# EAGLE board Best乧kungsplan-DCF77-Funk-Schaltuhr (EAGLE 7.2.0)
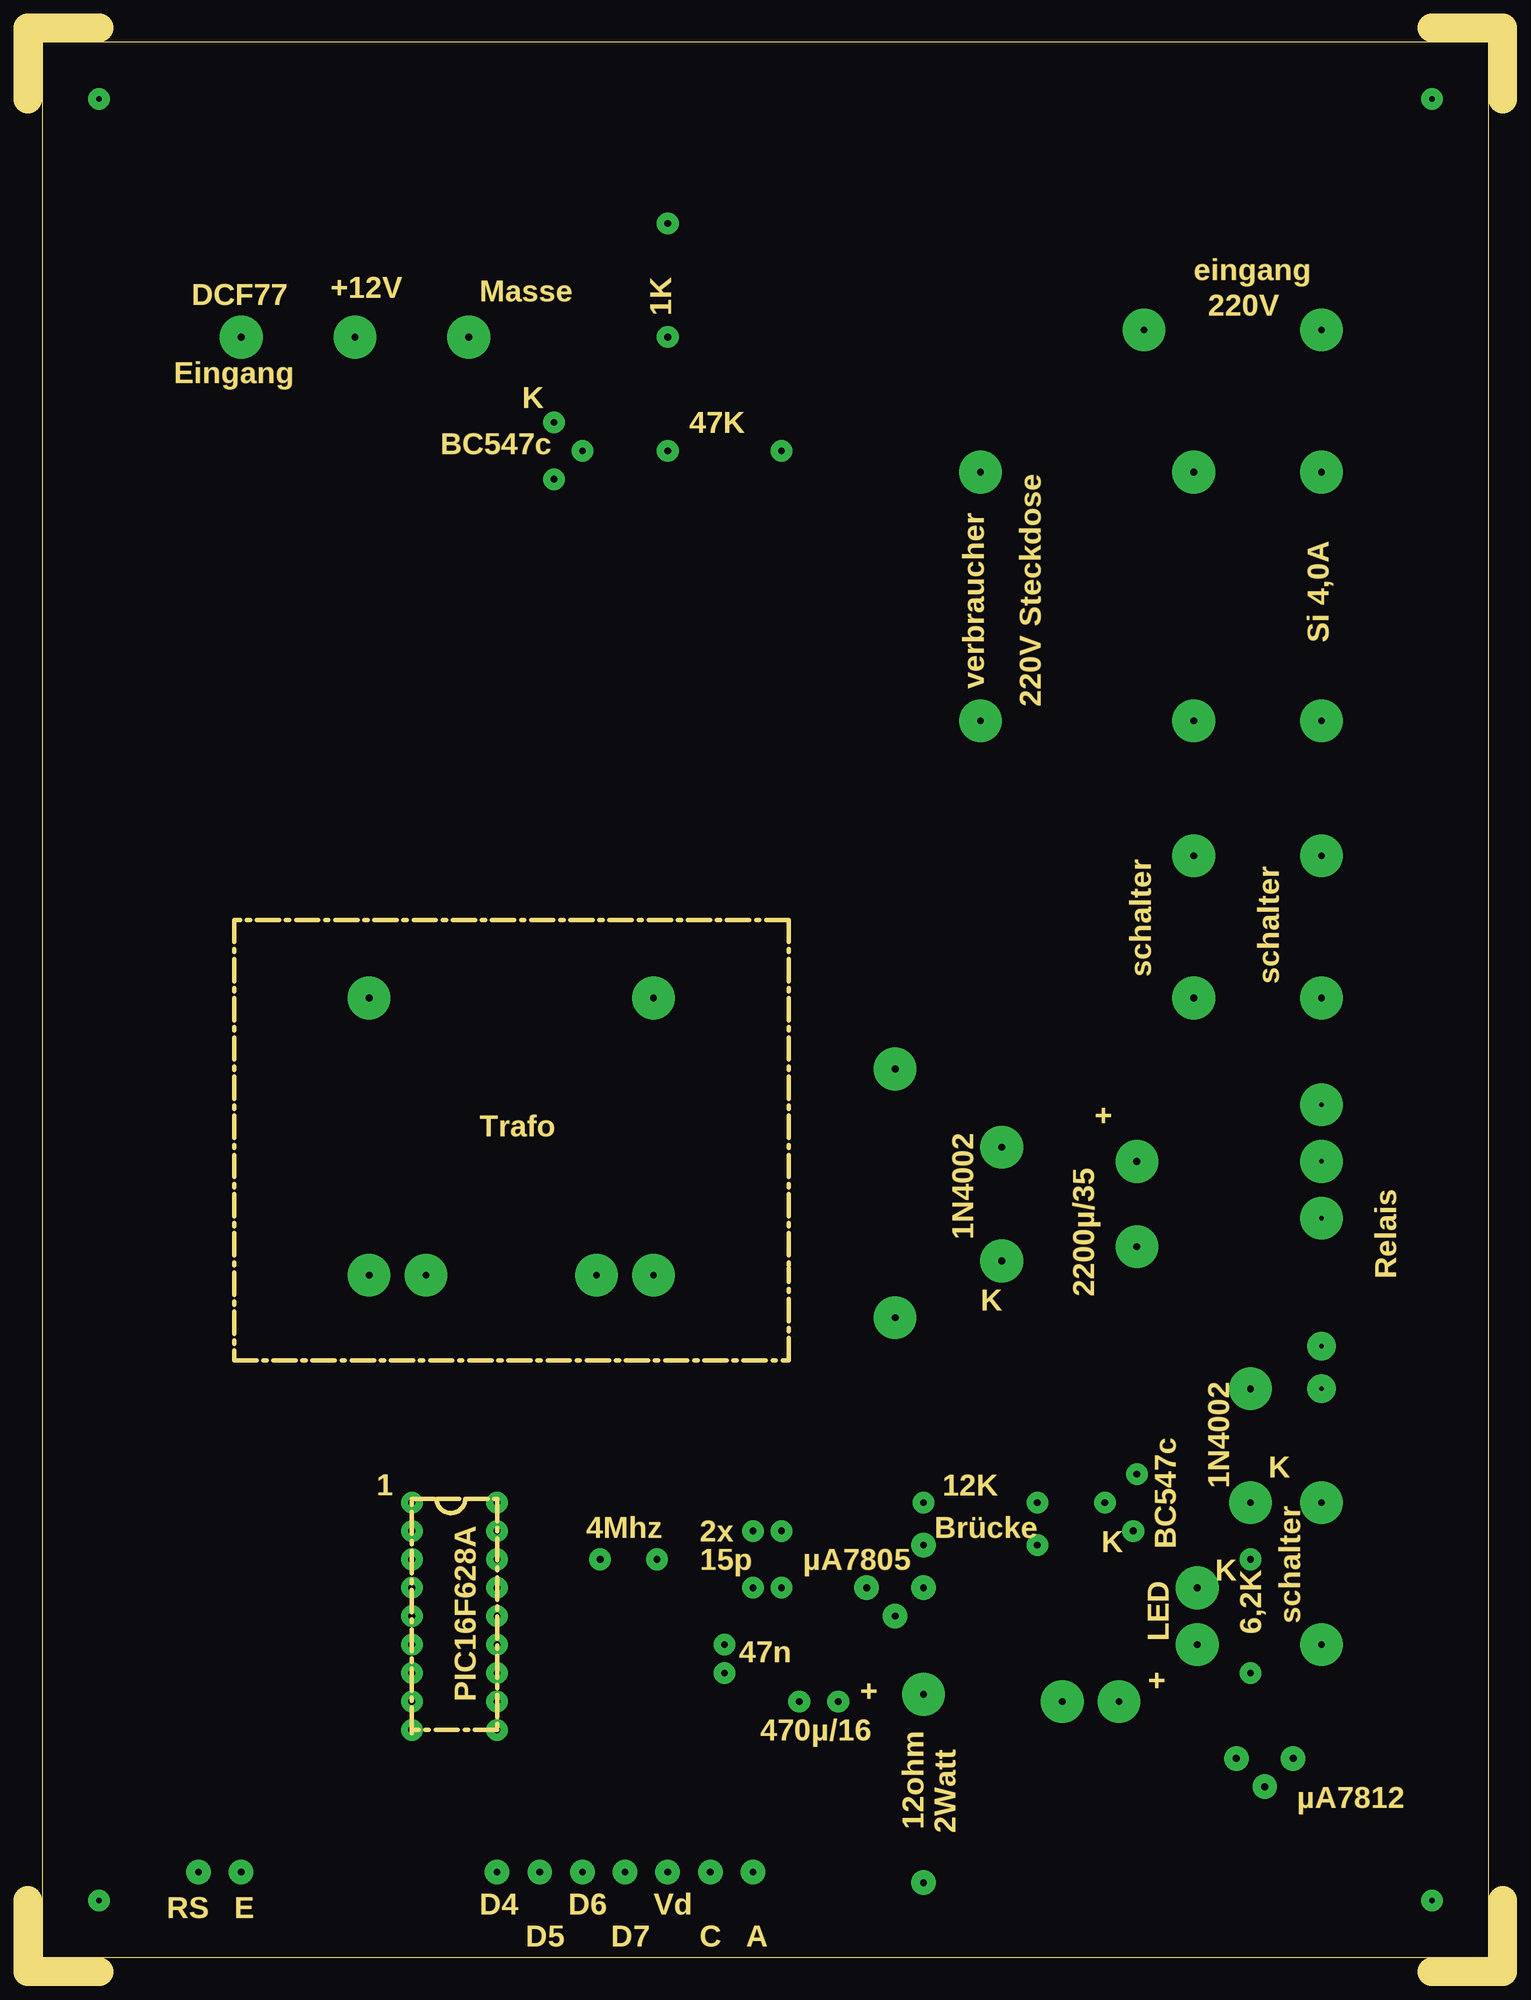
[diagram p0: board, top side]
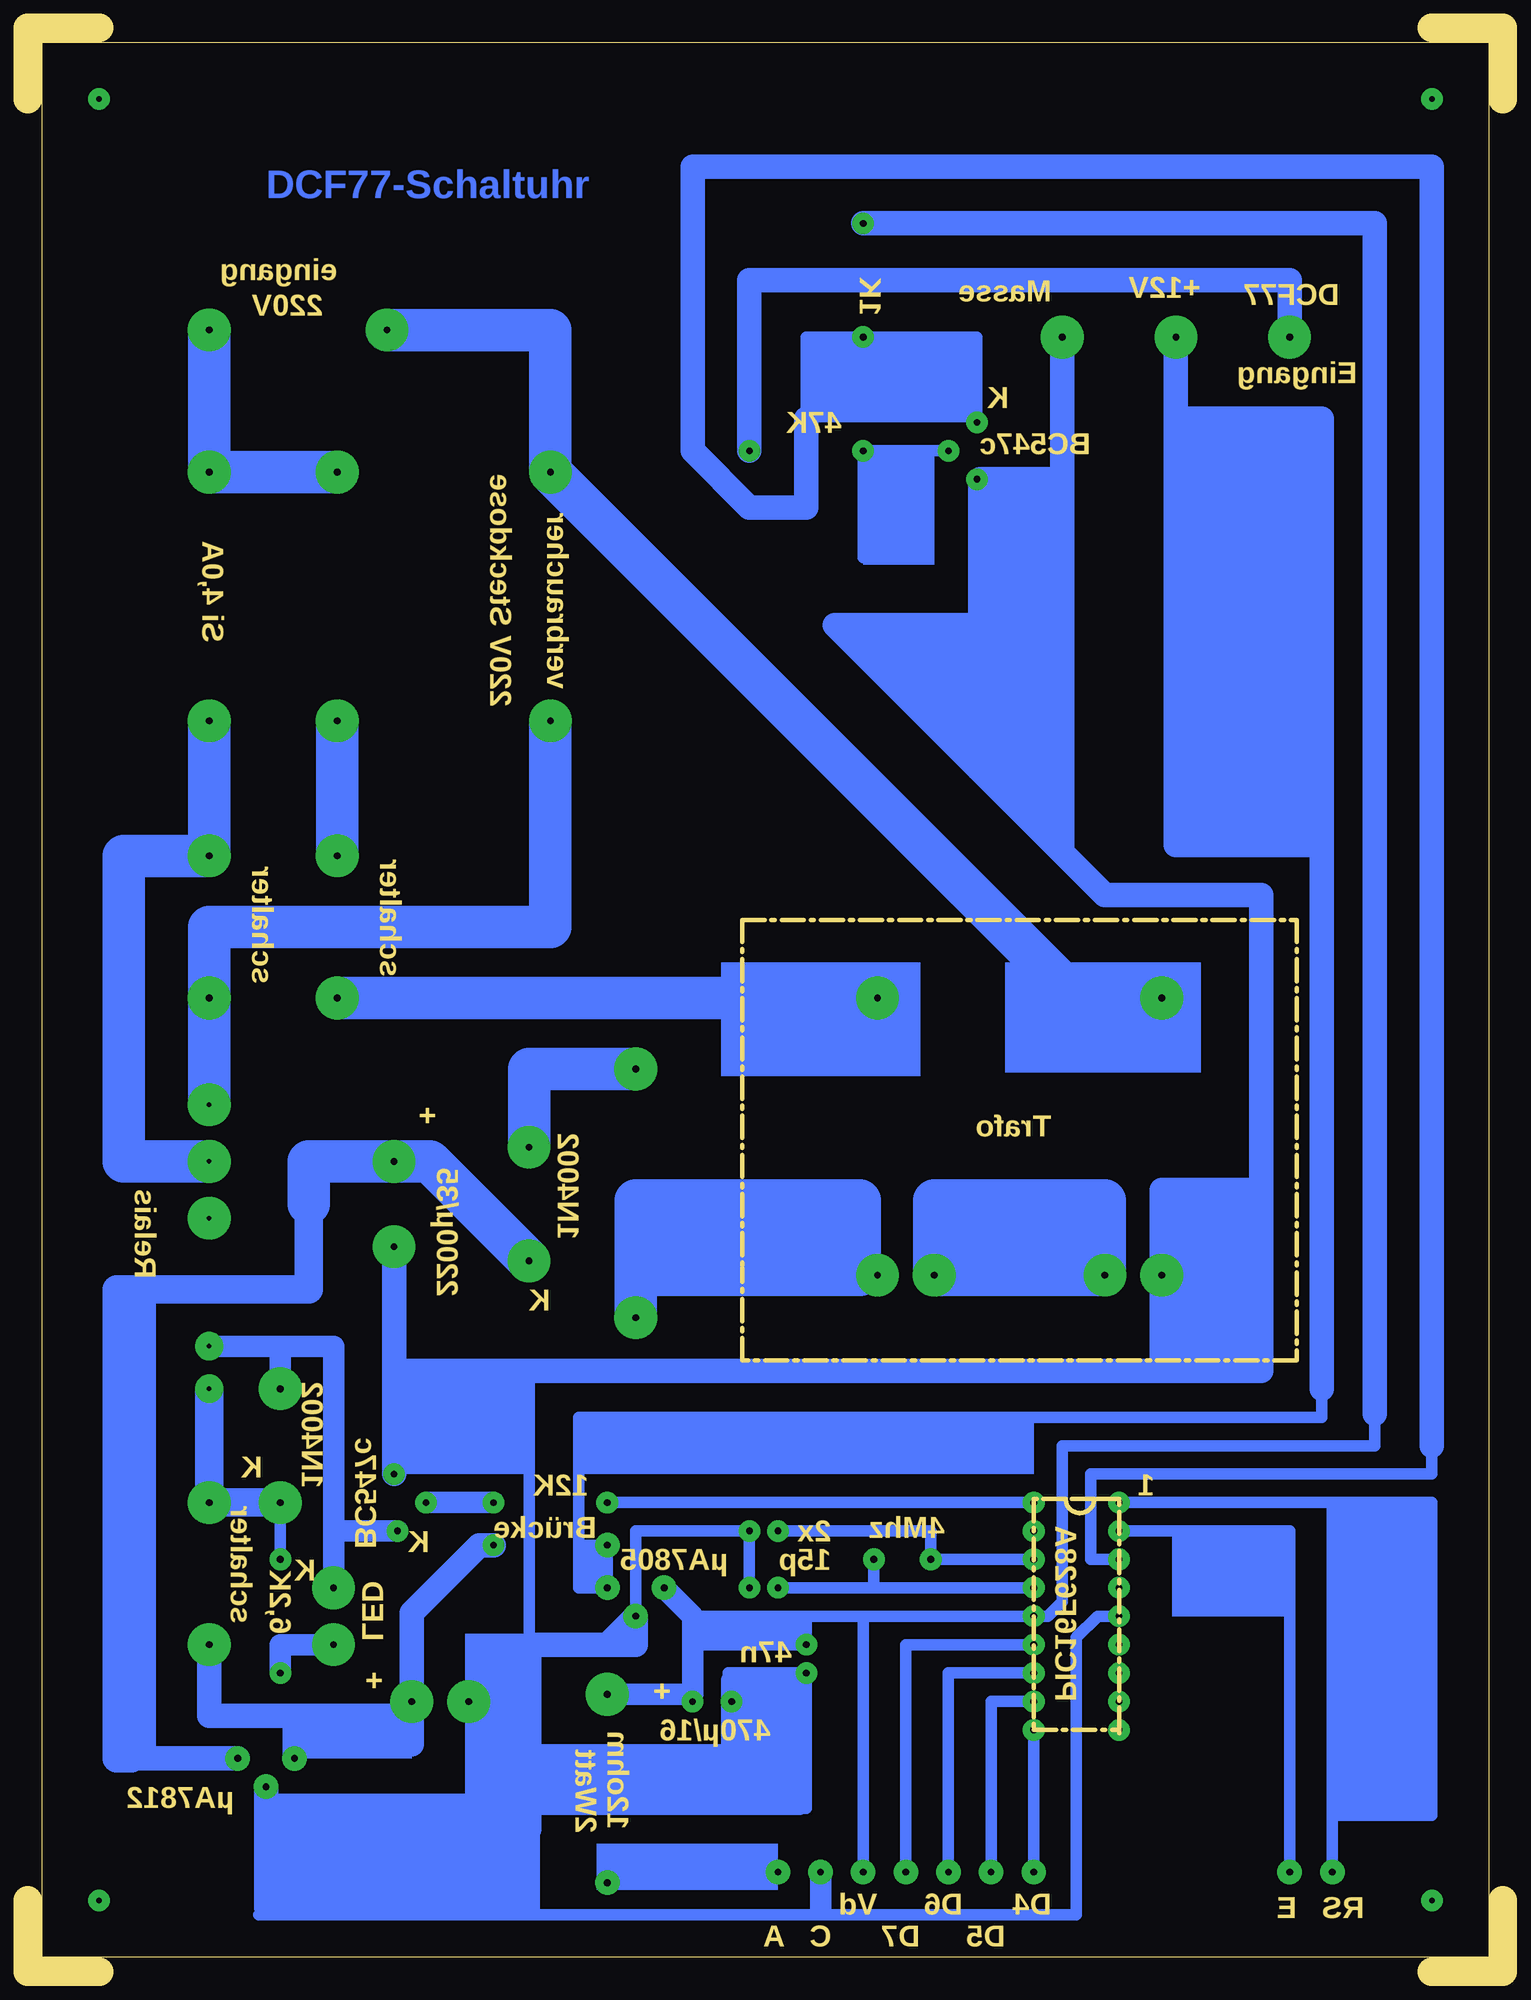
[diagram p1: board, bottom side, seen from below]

Size 131.76 x 173.67 mm. Coordinates in mm from the lower left corner, seen from the top.
Outline: 0,6.35 0,1.59 0,1.27 0,0 6.35,0
Outline: 131.76,6.35 131.76,0 125.41,0
Outline: 0,167.32 0,173.67 6.35,173.67
Outline: 131.76,167.32 131.76,173.67 125.41,173.67
Outline: 36.51,42.23 34.29,42.23 34.29,21.59
Outline: 36.51,42.23 39.05,42.23
Outline: 39.05,42.23 41.91,42.23 41.91,21.59 34.29,21.59
Outline: 34.29,21.59 34.29,21.27
Outline: 36.51,42.23 arc180 39.05,42.23
Outline: 1.27,1.27 130.49,1.27 130.49,172.4 1.27,172.4 1.27,1.27
Outline: 67.94,93.98 67.94,62.87 67.94,62.23 67.94,54.61 18.41,54.61 18.41,93.98 67.94,93.98
Copper layers (1*16): Top 0.035mm / dielectric 1.5mm / Bottom 0.035mm
Design rules "default": minimum track width 10mil, minimum drill 24mil, track to track 8mil, track to pad 8mil, pad to pad 8mil, via to via 8mil, smd to smd 8mil, copper to edge 40mil, drill to drill 8mil, minimum pad ring 10mil, minimum via ring 8mil, stop-mask expansion 4mil, vias tented up to drill 0mil, thermal gap 10mil

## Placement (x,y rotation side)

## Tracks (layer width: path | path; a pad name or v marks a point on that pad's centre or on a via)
S$1  (via drill 0.5 pad 1.93)
  other vias: 6.35,6.35
S$2  (via drill 0.5 pad 1.93)
  other vias: 6.35,167.32
S$3  (via drill 0.5 pad 1.93)
  other vias: 125.41,167.32
S$4  (via drill 0.5 pad 1.93)
  other vias: 125.41,6.35
S$5  (via drill 0.6 pad 1.93)
  other vias: 72.39,24.13
S$6  (via drill 0.6 pad 3.81)
  Bottom 3.81: v35.56,62.23 v50.8,62.23 50.8,68.9 35.56,68.9 v35.56,62.23
S$7  (via drill 0.6 pad 3.81)
  Bottom 3.81: v104.14,111.76 v104.14,99.69
S$8  (via drill 0.6 pad 3.81)
  Bottom 3.81: 77.47,61.91 77.47,62.23 57.47,62.23 57.47,68.9 77.47,68.9 77.47,61.91 | 77.47,61.91 v77.47,58.42
S$9  (via drill 0.6 pad 1.93, 0.6 pad 3.81)
  Bottom 2.184: v19.05,146.05 19.05,151.13 67.31,151.13 v67.31,135.89
S$10  (via drill 0.6 pad 3.81)
  other vias: 104.14,86.99
S$11  (via drill 0.6 pad 3.81)
  Bottom 3.81: v55.88,86.99 103.5,86.99
S$12  (via drill 0.6 pad 1.93, 0.6 pad 2.18, 0.6 pad 3.81)
  Bottom 2.184: v115.57,29.21 115.57,22.86 107.95,22.86 | v97.47,24.13 97.47,32.07 91.44,38.1 v90.17,38.1 | 107.95,22.86 v107.95,19.05 | 107.95,22.86 97.47,22.86 v97.47,24.13 | v97.47,24.13 97.47,20.32
S$13  (via drill 0.4 pad 3.81, 0.6 pad 3.81)
  Bottom 3.81: v85.09,111.76 85.09,93.34 115.57,93.34 v115.57,86.99 v115.57,77.47
S$14  (via drill 0.6 pad 2.18)
  Bottom 1.016: v64.77,8.89 79.06,8.89 v80.01,7.94
S$15  (via drill 0.6 pad 3.81)
  Bottom 3.81: v115.57,146.69 115.57,137.8 | 115.57,137.8 115.57,136.53 | v104.14,133.99 v115.57,133.99 115.57,137.8
S$16  (via drill 0.6 pad 1.93)
  Bottom 1.016: v34.29,41.91 15.56,41.91 | 15.56,41.91 15.24,41.91 15.24,13.97 | 15.24,13.97 15.24,8.89 | 15.56,41.91 6.35,41.91 6.35,13.97 15.24,13.97
S$17  (via drill 0.6 pad 1.93, 0.6 pad 2.18)
  Bottom 1.016: v34.29,39.37 19.05,39.37 v19.05,8.89
S$18  (via drill 0.6 pad 3.81)
  Bottom 3.81: v99.69,146.69 85.09,146.69 v85.09,133.99 38.1,86.99 v30.48,86.99
S$19  (via drill 0.6 pad 3.81)
  other vias: 55.88,62.23
S$20  (via drill 0.6 pad 1.93)
  other vias: 34.29,34.29
S$21  (via drill 0.6 pad 1.93)
  Bottom 1.016: v34.29,31.75 36.2,31.75 38.1,29.84 38.1,12.38
S$22  (via drill 0.6 pad 1.93)
  other vias: 34.29,29.21
S$24  (via drill 0.6 pad 1.93)
  other vias: 34.29,24.13
S$25  (via drill 0.6 pad 1.93)
  other vias: 34.29,21.59
S$26  (via drill 0.6 pad 1.93)
  Bottom 1.016: v41.91,41.91 v80.01,41.91
S$27  (via drill 0.6 pad 1.93)
  other vias: 41.91,39.37
S$28  (via drill 0.6 pad 1.93)
  Bottom 1.016: v41.91,36.83 v51.12,36.83 51.12,39.37 v64.77,39.37
S$29  (via drill 0.6 pad 1.93)
  Bottom 1.016: v41.91,34.29 56.2,34.29 | 56.2,34.29 v56.2,36.83 | 56.2,34.29 v64.77,34.29
S$31  (via drill 0.6 pad 1.93, 0.6 pad 2.18)
  Bottom 1.016: v41.91,29.21 53.34,29.21 v53.34,8.89
S$32  (via drill 0.6 pad 1.93, 0.6 pad 2.18)
  Bottom 1.016: v41.91,26.67 49.53,26.67 v49.53,8.89
S$33  (via drill 0.6 pad 1.93, 0.6 pad 2.18)
  Bottom 1.016: v41.91,24.13 45.72,24.13 v45.72,8.89
S$34  (via drill 0.6 pad 1.93, 0.6 pad 2.18)
  Bottom 1.016: v41.91,21.59 v41.91,8.89
S$35  (via drill 0.6 pad 1.93, 0.6 pad 2.18)
  Bottom 1.016: 62.23,24.45 v62.23,26.67 69.21,26.67 69.21,24.13 | 62.23,24.45 62.23,24.13 v68.9,24.13 | v67.31,34.29 v67.31,39.37 77.47,39.37 v77.47,31.75 | 86.99,29.21 86.99,53.34 | 86.99,13.02 86.99,5.08 86.68,5.08 | 86.68,5.08 38.1,5.08 38.1,12.06 | 86.68,5.08 111.12,5.08 | 62.23,24.45 62.23,14.61 69.21,14.61
  Bottom 1.93: 68.9,19.68 v68.9,24.13 68.9,26.04 | 68.9,19.68 68.9,19.37 86.68,19.37 | 68.9,19.68 68.9,14.92 69.21,14.92 | 86.99,29.21 86.99,24.13 | 69.21,14.92 86.99,14.92 | 69.21,14.92 62.87,14.92
  Bottom 2.184: 110.49,13.97 110.49,12.7 86.99,12.7 86.99,13.02 86.99,14.92 86.99,29.21 80.96,29.21 | 110.49,13.97 v110.49,16.51 | 80.96,29.21 80.01,29.21 v77.47,31.75 77.47,29.21 80.96,29.21 | 110.49,13.97 110.49,5.71
S$36  (via drill 0.6 pad 3.81)
  Bottom 3.81: v77.47,80.64 86.99,80.64 v86.99,73.66
S$37  (via drill 0.6 pad 1.93)
  other vias: 34.29,26.67
S$38  (via drill 0.6 pad 3.81)
  Bottom 2.184: v92.39,24.13 87.31,24.13
S$39  (via drill 0.6 pad 1.93)
  Bottom 1.93: v90.17,41.91 v96.2,41.91
S$40  (via drill 0.6 pad 2.18, 0.6 pad 3.81)
  Bottom 2.184: v113.03,19.05 122.87,19.05
  Bottom 2.54: 106.05,72.39 v99.06,72.39 | 106.68,68.58 106.68,60.96 123.83,60.96 123.83,19.05 122.87,19.05 122.55,19.05
  Bottom 3.81: v86.99,63.5 95.88,72.39 98.42,72.39 | v99.06,72.39 98.42,72.39 | 98.42,72.39 106.05,72.39 106.68,72.39 106.68,68.58
S$42  (via drill 0.4 pad 3.81, 0.6 pad 3.81)
  Bottom 3.81: v115.57,72.39 123.19,72.39 123.19,99.69 v115.57,99.69 v115.57,111.76
S$43  (via drill 0.4 pad 3.81)
  other vias: 115.57,67.31
S$47  (via drill 0.4 pad 2.54, 0.6 pad 1.93, 0.6 pad 3.81)
  Bottom 1.016: v109.22,41.91 v109.22,36.83
  Bottom 2.54: v115.57,52.07 v115.57,41.91 v109.22,41.91
S$48  (via drill 0.6 pad 2.18)
  Bottom 1.016: 82.55,38.42 82.55,38.1 v80.01,38.1 v80.01,34.29 82.55,34.29 82.55,38.42 | 82.55,38.42 82.55,49.53 16.19,49.53
S$49  (via drill 0.4 pad 2.54, 0.6 pad 1.93, 0.6 pad 3.81)
  Bottom 1.93: v115.57,55.88 109.22,55.88 | 109.22,55.88 104.46,55.88 104.46,39.37 | 104.46,39.37 v98.74,39.37 | 109.22,55.88 v109.22,52.07 | v104.46,34.29 104.46,39.37
S$50  (via drill 0.6 pad 1.93, 0.6 pad 3.81)
  Bottom 1.93: v104.46,29.21 109.22,29.21 v109.22,26.67
S$52  (via drill 0.6 pad 2.18, 0.6 pad 3.81)
  Bottom 1.93: v74.93,34.29 72.39,31.75 72.39,24.77 v80.01,24.77
S$53  (via drill 0.6 pad 3.81)
  other vias: 39.37,146.05
S$55  (via drill 0.6 pad 3.81)
  Bottom 1.016: 16.19,52.07 16.19,49.53
  Bottom 2.184: 16.19,52.07 16.19,100.33 | 16.19,100.33 16.19,100.65 29.21,100.65 29.21,138.75 | 29.21,138.75 v29.21,146.05 | 16.19,100.33 16.19,138.75 29.21,138.75
S$56  (via drill 0.6 pad 2.18)
  other vias: 15.24,8.89
S$57  (via drill 0.6 pad 2.18)
  Bottom 1.016: 60.96,5.71 60.96,5.4
  Bottom 1.93: v60.96,8.89 60.96,5.71
S$59  (via drill 0.6 pad 1.93, 0.6 pad 3.81)
  Bottom 1.016: 21.59,78.1 21.59,83.19 | 21.59,78.1 21.59,77.79 | 21.59,71.12 21.59,78.1 | v30.48,62.23 30.48,62.55 | 39.69,146.05 39.37,146.05 39.37,133.35 | 39.37,133.35 39.37,125.73 | 39.37,125.73 39.37,100.33 | 39.37,125.73 46.99,125.73 | 39.37,133.35 40.01,133.35 | 46.67,133.35 v46.99,133.35
  Bottom 2.184: 99.06,53.66 v99.06,64.77 | 30.48,53.98 v30.48,62.23 | 30.48,53.66 99.06,53.66 | 99.06,53.66 v99.06,44.45 | v30.48,62.23 21.59,62.23 21.59,69.85 | 21.59,69.85 21.59,71.12 21.59,83.19 21.59,96.2 35.56,96.2 39.37,100.01 | 39.37,100.01 39.37,146.05 | 39.37,100.01 59.69,120.33 46.67,120.33 46.67,133.35 40.01,133.35 | v30.48,62.23 30.48,69.85 21.59,69.85 | 21.59,69.85 21.59,53.98 30.48,53.98 | 30.48,53.66 30.48,53.98 | 21.59,53.66 30.48,53.66
S$60  (via drill 0.6 pad 1.93)
  Bottom 1.016: v46.99,138.43 46.99,146.05 v57.15,146.05 62.23,146.05 62.23,138.75 | v34.29,36.83 36.83,36.83 36.83,44.45 6.35,44.45 6.35,46.99
  Bottom 2.184: 62.23,138.75 62.23,130.81 67.31,130.81 72.39,135.89 72.39,161.29 6.35,161.29 6.35,135.89 6.35,46.99
S$62  (via drill 0.6 pad 1.93)
  Bottom 1.016: v49.53,135.89 v57.15,135.89 57.15,126.36
S$68  (via drill 0.6 pad 1.93, 0.6 pad 2.18)
  Bottom 1.016: 57.15,31.75 v41.91,31.75 40.64,31.75 39.37,33.02 39.37,46.99 11.43,46.99 11.43,49.85 | 57.15,31.75 62.23,31.75 | 62.23,31.75 72.07,31.75 | 62.23,31.75 v62.23,29.21 72.07,29.21 | 57.15,31.75 v57.15,8.89 | v57.15,156.21 57.47,156.21
  Bottom 2.184: v57.15,156.21 11.43,156.21 11.43,111.12 11.43,49.85
(copper drawn outside any net)
  shapes: Bottom area x35

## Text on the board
Bottom: DCF77-Schaltuhr
Pads: AUF BESTÜCKUNGS-SEITE GESEHEN
Dimension: Trafo 1,0mm | µA7812 + µA7805 1,0mm | eingang | DCF77 | +12V | Masse | 1K | 220V | Eingang | K | 47K | BC547c | K | Si 4,0A | LED rot Low Current | verbraucher | 220V Steckdose | hier ohne Fassung | gezeichnet | schalter | schalter | + | Trafo | 1N4002 | Relais | 2200µ/35 | K | und µA7812 | 12K | K | 1N4002 | 1 | 4Mhz | 2x | Brücke | BC547c | K | 15p | µA7805 | K | schalter | 6,2K | LED | 47n | + | PIC16F628A | + | 470µ/16 | µA7812 | 12ohm | 2Watt | D4 | D6 | Vd | RS | E | D5 | D7 | C | A
tOrigins: Alles mit 0,8mm vorbohren ! | BC547C | Aufbohren: | Diode 1N4002 1,0mm | Sicherungshalter 1,5mm | Anschluß-Drähte 1,0mm | 4Stck. Befestigungsbohr... 3,2mm | Brücke 1,0mm | K | E | 5,6ohm 1,0mm | B | LED 1,0mm | Die 3 Wechsel-Schalt- | 1N4002 | Anschlüsse vom Relais 1,2mm | Leiterplatte: | 1,5mm dick | Cevausit | Katode | Anode | ACHTUNG: | Die eine Brücke nicht vergessen | Si 400mA | K | wie | Katode | Anode | immer an + Pol | IC's | 1 | Die Aussparung | Links oben ist | muß mit dem | immer PIN 1 | Bauelement | und dem Bestück- | Si 400mA | ungsplan | überein stimmen. | µA7805 | Eing. | Eing. | Ausg. | Eing. | 1000µ/35V | Masse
